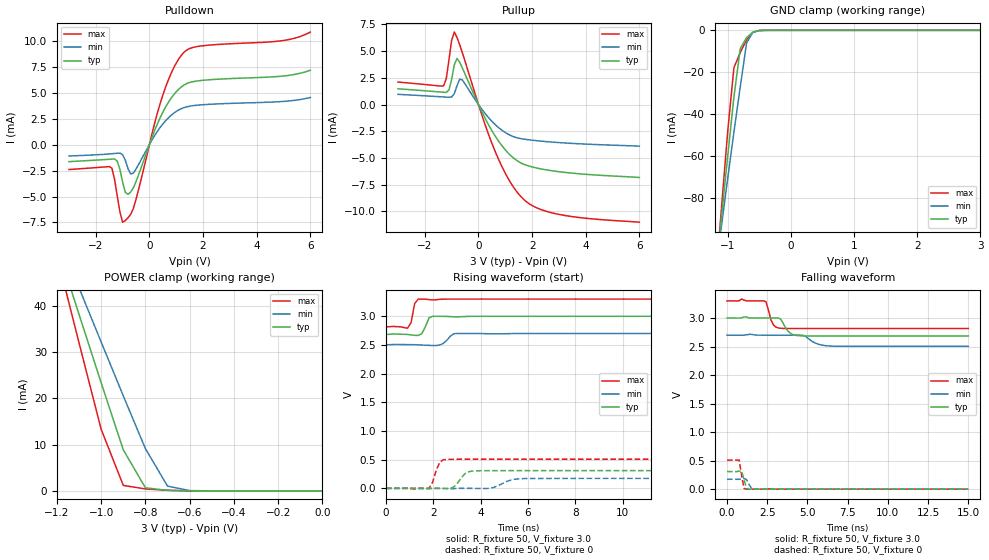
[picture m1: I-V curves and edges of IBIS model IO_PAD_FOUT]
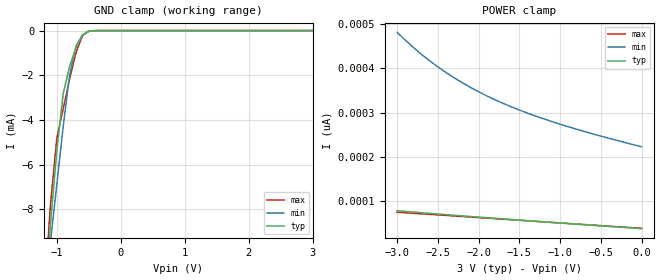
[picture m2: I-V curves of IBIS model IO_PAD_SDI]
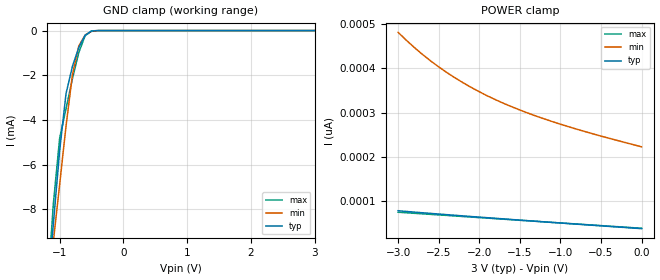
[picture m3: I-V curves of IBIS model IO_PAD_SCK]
[IBIS Ver]   3.2
[Comment Char]   |_char
[File name]   rx4111ce_3v.ibs
[File Rev]   1.0
[Date]   2019/10/04 4:25:01
[Source]
[Notes]
[Disclaimer]
This information is for modeling purposes only, and is not guaranteed.
Property of SEIKO EPSON Corp.,
unauthorized reproduction and/or distribution is strictly prohibited.
[Copyright]
Copyright 2019, SEIKO EPSON Corp.
[Component]   T5462W0A
Si_location Pin
Timing_location Pin
[Manufacturer]   SEIKO EPSON Corp.
| RX-4111CE
[Package]
R_pkg   267m   NA   NA
L_pkg   2.8nH   NA   NA
C_pkg   0.70pF   NA   NA
[Pin] signal_name   model_name
1   VDD   POWER
2   VBAT   POWER
3   DI   IO_PAD_SDI
4   FOUT   IO_PAD_FOUT
5   CLK   IO_PAD_SCK
6   DO   IO_PAD_SDO
7   CE   IO_PAD_CE
8   VIO   POWER
9   GND   GND
10   /INT   IO_PAD_XINT
| Models and submodels in the file (6): IO_PAD_FOUT (3-state), IO_PAD_SDI (Input), IO_PAD_SCK (Input), IO_PAD_SDO (3-state), IO_PAD_CE (Input), IO_PAD_XINT (Open_drain)
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[Model]   IO_PAD_FOUT
Model_type 3-state
Enable Active-High
Polarity Non-Inverting
Vmeas=1.50
C_comp   2.5p   2.0p   3.0p
[Temperature Range] 25   105   -40
[Voltage Range]   3.0   2.7   3.3
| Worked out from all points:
|   slope of the pulldown table from 0 to 0.45 V, typ, clamps not added: 158 ohm
|   slope of the pullup table from 0 to 0.45 V, typ, clamps not added: 202 ohm
|   GND clamp passes 1 mA (typ) near -0.60 V on its own axis
|   POWER clamp passes 1 mA (typ) near -0.80 V on its own axis
|   falling waveform, R_fixture 50, V_fixture 3.0: 20-80 % time 453ps typ, 696ps min, 319ps max; typ from 3 V to 2.69 V
|   falling waveform, R_fixture 50, V_fixture 0: 20-80 % time 184ps typ, 208ps min, 185ps max; typ from 0.309 V to 0 V
|   rising waveform, R_fixture 50, V_fixture 3.0: 20-80 % time 205ps typ, 279ps min, 132ps max; typ from 2.69 V to 3 V
|   rising waveform, R_fixture 50, V_fixture 0: 20-80 % time 365ps typ, 571ps min, 257ps max; typ from 0 V to 0.309 V
[Pullup]
-3V       1.471mA    952.6uA    2.104mA
-1.3V     1.147mA    709.8uA    1.738mA
-1.2V     1.13mA     694.5uA    2.414mA
-1.1V     1.366mA    679uA      4.16mA
-1V       2.339mA    705.4uA    6.008mA
-900mV    3.706mA    1.017mA    6.776mA
-800mV    4.313mA    1.748mA    6.271mA
-600mV    3.419mA    2.299mA    4.848mA
600mV     -2.854mA   -1.818mA   -4.245mA
1.6V      -5.487mA   -3.2mA     -8.66mA
2.9V      -6.251mA   -3.543mA   -10.23mA
6V        -6.823mA   -3.898mA   -11.01mA
[Pulldown]
-3V       -1.645mA   -1.105mA   -2.404mA
-1.4V     -1.401mA   -881.9uA   -2.281mA
-1.2V     -1.594mA   -838.2uA   -4.933mA
-1V       -3.61mA    -971.9uA   -7.472mA
-800mV    -4.793mA   -2.307mA   -7.046mA
-600mV    -4.172mA   -2.75mA    -6.158mA
500mV     3.112mA    1.977mA    4.757mA
900mV     4.773mA    3.003mA    7.349mA
1.3V      5.744mA    3.563mA    8.902mA
2V        6.182mA    3.832mA    9.508mA
5V        6.596mA    4.15mA     10.01mA
6V        7.149mA    4.527mA    10.82mA
[GND Clamp]
-3V       -666mA     -547.8mA   -822.2mA
-1.2V     -119.6mA   -117.1mA   -123.7mA
-1.1V     -89.89mA   -93.83mA   -85.8mA
-1V       -60.42mA   -70.86mA   -48.73mA
-900mV    -31.79mA   -48.51mA   -17.79mA
-800mV    -8.762mA   -26.99mA   -10.57mA
-700mV    -3.482mA   -6.087mA   -4.558mA
-600mV    -875.1uA   -938.3uA   -964.6uA
-500mV    -86.79uA   -136.7uA   -53.06uA
-400mV    -4.756uA   -14.79uA   -1.084uA
3V        37.81pA    65.05nA    23.86pA
[POWER Clamp]
-3V       323.7mA    269.5mA    395.6mA
-1.2V     53.06mA    55.67mA    50.96mA
-1.1V     38.19mA    43.92mA    32.03mA
-1V       23.39mA    32.21mA    13.33mA
-900mV    8.898mA    20.56mA    1.192mA
-800mV    679.8uA    9.149mA    426.2uA
-700mV    116.6uA    1.034mA    140.4uA
-600mV    22.63uA    76.12uA    22.74uA
0V        37.92pA    763.7pA    29.64pA
[Falling Waveform]
R_fixture=50
V_fixture=3.0
V_fixture_min=2.7
V_fixture_max=3.3
0s        3V         2.7V       3.3V
909.1ps   3.003V     2.699V     3.333V
2.424ns   3V         2.7V       3.286V
2.727ns   3V         2.7V       2.971V
2.879ns   3V         2.7V       2.883V
3.333ns   2.982V     2.7V       2.82V
3.788ns   2.77V      2.7V       2.817V
4.394ns   2.692V     2.7V       2.817V
6.364ns   2.685V     2.511V     2.816V
15ns      2.685V     2.505V     2.816V
[Falling Waveform]
R_fixture=50
V_fixture=0
V_fixture_min=0
V_fixture_max=0
0s        308.8mV    173.5mV    508.3mV
606.1ps   306.9mV    172.2mV    509.2mV
757.6ps   317.4mV    172.5mV    510.2mV
909.1ps   318.5mV    177.7mV    238.4mV
1.061ns   167.4mV    186mV      11.86mV
1.212ns   14.15mV    167.8mV    329.8uV
1.364ns   1.997mV    84.14mV    10.39uV
1.515ns   201.5uV    15.32mV    -15.29uV
1.818ns   11.09uV    1.012mV    -15.97uV
15ns      0V         0V         621.2nV
[Rising Waveform]
R_fixture=50
V_fixture=3.0
V_fixture_min=2.7
V_fixture_max=3.3
0s        2.685V     2.505V     2.816V
909.1ps   2.683V     2.506V     2.791V
1.061ns   2.675V     2.505V     2.887V
1.212ns   2.668V     2.505V     3.221V
1.364ns   2.666V     2.502V     3.299V
1.515ns   2.697V     2.499V     3.299V
1.818ns   2.971V     2.493V     3.291V
1.97ns    3V         2.491V     3.285V
3.03ns    2.991V     2.7V       3.3V
15ns      3V         2.7V       3.3V
[Rising Waveform]
R_fixture=50
V_fixture=0
V_fixture_min=0
V_fixture_max=0
0s        0V         0V         0V
1.818ns   -8.601mV   102.5uV    633.1uV
2.273ns   -361.6uV   -684.4uV   455.5mV
2.576ns   -2.263mV   -3.519mV   505.4mV
2.879ns   27.32mV    -4.664mV   507.4mV
3.333ns   253.3mV    3.654uV    508.1mV
3.788ns   305.3mV    -550.9uV   508.3mV
4.394ns   308.2mV    1.863mV    508.3mV
5.758ns   308.8mV    169.3mV    508.3mV
15ns      308.8mV    173.5mV    508.3mV
[Ramp]
R_load=50
dV/dt_r   1.853E-1/3.478E-10   1.041E-1/5.635E-10   3.050E-1/2.294E-10
dV/dt_f   1.891E-1/4.362E-10   1.172E-1/6.888E-10   2.901E-1/2.838E-10
|[End   IO_PAD_FOUT
[Model]   IO_PAD_SDI
Model_type Input
Enable Active-High
Polarity Non-Inverting
Vinh=2.64
Vinl=0.54
C_comp   2.5p   2.0p   3.0p
[Temperature Range] 25   105   -40
[Voltage Range]   3.0   2.7   3.3
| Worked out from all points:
|   GND clamp passes 1 mA (typ) near -0.73 V on its own axis
[GND Clamp]
-3V       -73.52mA   -59.85mA   -89.54mA
-1.2V     -12.05mA   -12.06mA   -12.02mA
-1.1V     -8.699mA   -9.474mA   -7.793mA
-1V       -5.361mA   -6.879mA   -4.813mA
-900mV    -2.819mA   -4.28mA    -3.497mA
-800mV    -1.604mA   -1.983mA   -2.157mA
-700mV    -762.3uA   -688.3uA   -983.1uA
-600mV    -207.7uA   -196.5uA   -228.8uA
-500mV    -21.87uA   -34.46uA   -13.49uA
-300mV    -47nA      -340.4nA   -3.539nA
3V        38.75pA    237.5pA    36.05pA
[POWER Clamp]
-3V       79.16pA    481pA      75.69pA
-2.9V     77.56pA    463.4pA    74.6pA
-2.7V     74.53pA    431.2pA    72.15pA
-2.5V     71.72pA    403.2pA    69.7pA
-2.4V     70.27pA    390.5pA    68.6pA
-2.2V     67.5pA     367.5pA    66.08pA
-1.9V     63.37pA    337.9pA    62.53pA
-1.7V     60.73pA    321.1pA    60.01pA
-1.5V     58.05pA    306.1pA    57.57pA
-1.1V     52.71pA    280pA      52.82pA
-600mV    46.36pA    252.5pA    46.82pA
0V        38.75pA    223.1pA    39.63pA
[Model]   IO_PAD_SCK
Model_type Input
Enable Active-High
Polarity Non-Inverting
Vinh=2.64
Vinl=0.54
C_comp   2.5p   2.0p   3.0p
[Temperature Range] 25   105   -40
[Voltage Range]   3.0   2.7   3.3
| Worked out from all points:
|   GND clamp passes 1 mA (typ) near -0.73 V on its own axis
[GND Clamp]
-3V       -73.52mA   -59.85mA   -89.54mA
-1.2V     -12.05mA   -12.06mA   -12.02mA
-1.1V     -8.699mA   -9.474mA   -7.793mA
-1V       -5.361mA   -6.879mA   -4.813mA
-900mV    -2.819mA   -4.28mA    -3.497mA
-800mV    -1.604mA   -1.983mA   -2.157mA
-700mV    -762.3uA   -688.3uA   -983.1uA
-600mV    -207.7uA   -196.5uA   -228.8uA
-500mV    -21.87uA   -34.46uA   -13.49uA
-300mV    -47nA      -340.4nA   -3.539nA
3V        38.74pA    237.5pA    36.06pA
[POWER Clamp]
-3V       79.15pA    481pA      75.72pA
-2.9V     77.55pA    463.4pA    74.62pA
-2.7V     74.53pA    431.2pA    72.17pA
-2.5V     71.71pA    403.2pA    69.72pA
-2.3V     68.86pA    378.6pA    67.28pA
-2.2V     67.49pA    367.5pA    66.1pA
-1.9V     63.36pA    337.9pA    62.55pA
-1.7V     60.73pA    321.1pA    60.03pA
-1.5V     58.04pA    306.1pA    57.59pA
-1.1V     52.71pA    280pA      52.84pA
-600mV    46.36pA    252.5pA    46.84pA
0V        38.74pA    223.1pA    39.64pA
